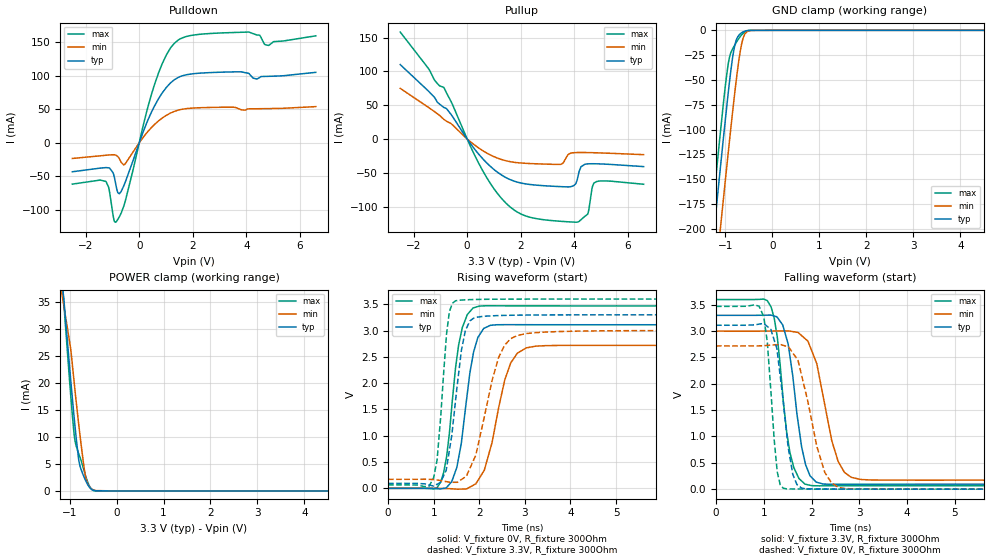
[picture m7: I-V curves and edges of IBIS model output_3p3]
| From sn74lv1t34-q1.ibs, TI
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[Model]   output_3p3
Model_type   Output
Polarity   Non-Inverting
Vmeas = 1.5
Vref = 0
Cref = 15pF
Rref = 1000000
|   typ   min   max
C_comp   4.947pF   4.835pF   5.043pF
[Voltage Range]   3.3   3   3.6
[Temperature Range]   27   125   -40
[Pullup Reference]   3.3   3   3.6
[Pulldown Reference]   0   0   0
[Power Clamp Reference]   3.3   3   3.6
[GND Clamp Reference]   0   0   0
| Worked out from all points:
|   slope of the pulldown table from 0 to 0.495 V, typ, clamps not added: 10.1 ohm
|   slope of the pullup table from 0 to 0.495 V, typ, clamps not added: 19.6 ohm
|   GND clamp passes 1 mA (typ) near -0.59 V on its own axis
|   POWER clamp passes 1 mA (typ) near -0.60 V on its own axis
|   falling waveform, V_fixture 3.3V, R_fixture 300Ohm: 20-80 % time 283ps typ, 398ps min, 251ps max; typ from 3.3 V to 0.094 V
|   rising waveform, V_fixture 0V, R_fixture 300Ohm: 20-80 % time 298ps typ, 430ps min, 263ps max; typ from 0 V to 3.11 V
|   rising waveform, V_fixture 3.3V, R_fixture 300Ohm: 20-80 % time 269ps typ, 455ps min, 181ps max; typ from 0.094 V to 3.3 V
|   falling waveform, V_fixture 0V, R_fixture 300Ohm: 20-80 % time 245ps typ, 413ps min, 168ps max; typ from 3.11 V to 0 V
[Pulldown]
|   Voltage   I(typ)   I(min)   I(max)
-2.5V     -43.18mA   -23.37mA   -61.62mA
-1.25V    -37.01mA   -18.58mA   -57.53mA
-977.5mV  -44.66mA   -17.83mA   -108.2mA
-851.5mV  -66.87mA   -18.96mA   -117.3mA
-746.5mV  -76.02mA   -23.35mA   -110.5mA
-547mV    -61.15mA   -32.26mA   -90.4mA
576.5mV   55.38mA    27.5mA     87.6mA
1.018V    82.74mA    41.05mA    131.3mA
1.49V     98.08mA    49.01mA    154mA
4.104V    103mA      50.58mA    165mA
4.84V     99.09mA    50.98mA    145.2mA
6.593V    105mA      53.91mA    159.4mA
[GND Clamp]
|   Voltage   I(typ)   I(min)   I(max)
-2.5V     -817.8mA   -872.3mA   -789.1mA
-1.303V   -231.2mA   -292.1mA   -196.1mA
-1.23V    -196.2mA   -257.3mA   -160.8mA
-1.125V   -146.7mA   -208.1mA   -111.2mA
-1.062V   -117.5mA   -178.9mA   -82.22mA
-946mV    -65.86mA   -126.2mA   -35.86mA
-830.5mV  -22.76mA   -75.49mA   -17.36mA
-767.5mV  -9.785mA   -49.8mA    -12.22mA
-694mV    -3.965mA   -24.23mA   -6.893mA
-589mV    -891.1uA   -3.999mA   -1.764mA
-431.5mV  -12.85uA   -82.5uA    -10.97uA
8V        0A         0A         0A
[Pullup]
|   Voltage   I(typ)   I(min)   I(max)
-2.5V     110mA      74.9mA     158.1mA
-872.5mV  46.71mA    29.17mA    76.33mA
702.5mV   -34.17mA   -20.06mA   -55.22mA
1.805V    -62.92mA   -34.63mA   -106.3mA
3.495V    -70.37mA   -37.38mA   -121.6mA
3.968V    -69.17mA   -20.26mA   -122.8mA
4.115V    -59.51mA   -19.94mA   -122.8mA
4.252V    -40.97mA   -19.89mA   -119.3mA
4.503V    -36.74mA   -20.02mA   -111mA
4.661V    -36.53mA   -20.17mA   -73.41mA
4.745V    -36.55mA   -20.26mA   -64.8mA
6.593V    -40.77mA   -23.12mA   -66.88mA
[POWER Clamp]
|   Voltage   I(typ)   I(min)   I(max)
-2.5V     144.5mA    117mA      177mA
-1.219V   42.82mA    39.69mA    46.86mA
-1.125V   35.89mA    34.5mA     35.22mA
-977.5mV  20.83mA    26.44mA    18.04mA
-914.5mV  14.77mA    21.23mA    11.56mA
-883mV    11.92mA    18.58mA    9.292mA
-799mV    5.487mA    11.92mA    6.762mA
-715mV    3.079mA    5.916mA    4.489mA
-662.5mV  2.013mA    2.787mA    2.926mA
-589mV    837.6uA    921.4uA    1.128mA
-494.5mV  114.2uA    194.6uA    87.23uA
8V        0A         0A         0A
[Ramp]
R_load = 300
|   typ   min   max
dV/dt_r   1.86701/2.97801e-10   1.63117/4.29678e-10   2.08197/2.62916e-10
dV/dt_f   1.92339/2.82985e-10   1.69703/3.98282e-10   2.12049/2.514e-10
[Falling Waveform]
V_fixture = 3.3V
V_fixture_min = 3V
V_fixture_max = 3.6V
R_fixture = 300Ohm
C_fixture = 0F
|   Time   V(typ)   V(min)   V(max)
0s        3.3V       3V         3.6V
1.154ns   3.303V     3.001V     3.457V
1.282ns   3.263V     3.003V     2.899V
1.481ns   2.851V     3.004V     1.073V
1.548ns   2.521V     2.999V     692.6mV
1.863ns   517.6mV    2.859V     95.81mV
2.11ns    130.4mV    2.382V     64.36mV
2.559ns   93.23mV    522mV      64.97mV
2.834ns   93.79mV    223.6mV    65.5mV
15ns      94.34mV    171.6mV    65.84mV
[Rising Waveform]
V_fixture = 0V
V_fixture_min = 0V
V_fixture_max = 0V
R_fixture = 300Ohm
C_fixture = 0F
|   Time   V(typ)   V(min)   V(max)
0s        954.7nV    1.301uV    430.7nV
1.075ns   -7.226mV   24.91uV    13.43mV
1.282ns   14.79mV    -4.189mV   590.9mV
1.397ns   128.6mV    -8.874mV   1.554V
1.628ns   1.017V     -13.82mV   3.059V
1.793ns   2.191V     23.38mV    3.36V
2ns       2.912V     191.2mV    3.467V
2.689ns   3.113V     2.384V     3.471V
3.034ns   3.113V     2.672V     3.47V
15ns      3.112V     2.719V     3.47V
[Rising Waveform]
V_fixture = 3.3V
V_fixture_min = 3V
V_fixture_max = 3.6V
R_fixture = 300Ohm
C_fixture = 0F
|   Time   V(typ)   V(min)   V(max)
0s        94.34mV    171.6mV    65.84mV
1ns       43.1mV     166.4mV    202mV
1.075ns   77.89mV    157.9mV    541.9mV
1.282ns   382.8mV    127.1mV    2.935V
1.481ns   1.681V     115.3mV    3.567V
1.608ns   2.623V     167.7mV    3.581V
1.793ns   3.183V     377.2mV    3.589V
2.424ns   3.286V     2.487V     3.598V
2.834ns   3.294V     2.908V     3.599V
15ns      3.3V       3V         3.6V
[Falling Waveform]
|Gnd
V_fixture = 0V
V_fixture_min = 0V
V_fixture_max = 0V
R_fixture = 300Ohm
C_fixture = 0F
|   Time   V(typ)   V(min)   V(max)
0s        3.112V     2.719V     3.47V
1ns       3.147V     2.724V     3.276V
1.075ns   3.088V     2.729V     2.786V
1.282ns   2.614V     2.743V     329.4mV
1.409ns   1.649V     2.73V      17.99mV
1.51ns    803mV      2.703V     4.982mV
1.695ns   85.9mV     2.473V     3.495mV
2.279ns   3.002mV    314.4mV    1.041mV
2.559ns   1.781mV    36.9mV     569.7uV
15ns      463nV      1.302uV    432.5nV
